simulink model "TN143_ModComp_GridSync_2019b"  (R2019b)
settings: Solver=VariableStepAuto  StartTime=0.0  StopTime=0.1  RelTol=1e-3
model workspace (MAT data in the model file):
  CTRLPERIOD = 5e-05
  global_can_baud_rate = 1000000
  global_cycle_delay = 1e-05
  global_ip_addresses : object (value not decoded)
undefined symbols (not defined in the file): A, AXI4, C, code, HLS, N, Stream, xc7z030fbg676
libraries: ModelComposer x102

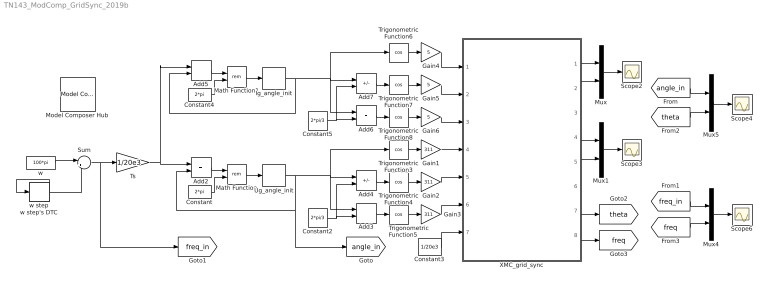
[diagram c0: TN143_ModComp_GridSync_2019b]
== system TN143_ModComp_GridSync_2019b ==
  Add{2..3,5..6} (4 alike) : Sum
  Add4 : Sum  Inputs=+-
  Add7 : Sum  Inputs=+-
  Constant : Constant  Value=2*pi  OutDataTypeStr=single
  Constant2 : Constant  Value=2*pi/3  OutDataTypeStr=single
  Constant3 : Constant  Value=1/20e3  OutDataTypeStr=single
  Constant4 : Constant  Value=2*pi  OutDataTypeStr=single
  Constant5 : Constant  Value=2*pi/3  OutDataTypeStr=single
  Gain1 : Gain  Gain=311
  Gain2 : Gain  Gain=311
  Gain3 : Gain  Gain=311
  Gain4 : Gain  Gain=5
  Gain5 : Gain  Gain=5
  Gain6 : Gain  Gain=5
  Ig_angle_init : Delay  DelayLength=1  InitialCondition=pi/2-pi/3
  Math Function : Math  Operator=rem
  Math Function1 : Math  Operator=rem
  Model Composer Hub : ModelComposer/Model Composer Hub  CodeGeneration=off  SubsystemName=XMC_grid_sync  TargetDirectory=C:/XMC/TN143/generated/code  ExportType=HLS C++ code  IpVendor=xilinx.com  IpLibrary=hls  IpVersion=1.0  IpHWLanguage=Verilog  AieCompilerOptions={}  CreateTestbench=off  TestbenchStackSize=10  RunAieSim=off  AieSimTimeout=50000  LaunchVitisAnalyzer=off  RunX86Sim=off  X86SimTimeout=10  ProjDevice=xc7z030fbg676-3  ProjDevicePart=xc7z030fbg676-3  SamplePeriod=-1  ClockFrequency=250  DataPathParallelism=1
  Mux{,1,4..5} (4 alike) : Mux  Inputs=2
  Scope{2..4,6} (4 alike) : Scope
  Sum : Sum  Inputs=|++
  Trigonometric Function{3..8} (6 alike) : Trigonometry  Operator=cos
  Ts : Gain  Gain=1/20e3
  Ug_angle_init : Delay  DelayLength=1  InitialCondition=0
  XMC_grid_sync : Subsystem  mask{PLL_KP=5, PLL_KI=2, FREQ=50}
      mask prompts: PLL_KP "PLL kp"; PLL_KI "PLL ki"; FREQ "PLL frequency(Hz)"
  w : Constant  Value=100*pi  OutDataTypeStr=single  SampleTime=1/20e3
  w step : Step  Time=0.02  After=10*pi
  w step's DTC : DataTypeConversion  OutDataTypeStr=single
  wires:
  Trigonometric Function4/1 -> Gain2/1
  Add2/1 -> Math Function/1
  Trigonometric Function3/1 -> Gain1/1
  Gain1/1 -> XMC_grid_sync/4(Ug_A)
  Gain3/1 -> XMC_grid_sync/6(Ug_C)
  Gain2/1 -> XMC_grid_sync/5(Ug_B)
  Constant2/1 -> Add4/2, Add3/2
  Add4/1 -> Trigonometric Function4/1
  Add3/1 -> Trigonometric Function5/1
  Math Function/1 -> Ug_angle_init/1
  Constant/1 -> Math Function/2
  Trigonometric Function5/1 -> Gain3/1
  Constant3/1 -> XMC_grid_sync/7(Ts)
  Gain6/1 -> XMC_grid_sync/3(Ig_C)
  Gain5/1 -> XMC_grid_sync/2(Ig_B)
  Gain4/1 -> XMC_grid_sync/1(Ig_A)
  XMC_grid_sync/1(Ig_d) -> Mux/1
  XMC_grid_sync/2(Ig_q) -> Mux/2
  Mux/1 -> Scope2/1
  XMC_grid_sync/4(Ug_d) -> Mux1/1
  XMC_grid_sync/5(Ug_q) -> Mux1/2
  Mux1/1 -> Scope3/1
  Ts/1 -> Add5/1, Add2/1
  Trigonometric Function8/1 -> Gain6/1
  Ig_angle_init/1 -> Trigonometric Function6/1, Add7/1, Add6/1, Add5/2
  Constant5/1 -> Add7/2, Add6/2
  Add7/1 -> Trigonometric Function7/1
  Constant4/1 -> Math Function1/2
  Add6/1 -> Trigonometric Function8/1
  Add5/1 -> Math Function1/1
  Trigonometric Function7/1 -> Gain5/1
  Trigonometric Function6/1 -> Gain4/1
  Math Function1/1 -> Ig_angle_init/1
  w/1 -> Sum/1
  Sum/1 -> Ts/1, [freq_in]
  Ug_angle_init/1 -> Trigonometric Function3/1, Add4/1, Add3/1, [angle_in], Add2/2
  XMC_grid_sync/7(theta) -> [theta]
  XMC_grid_sync/8(freq) -> [freq]
  [freq_in] -> Mux4/1
  [freq] -> Mux4/2
  [angle_in] -> Mux5/1
  [theta] -> Mux5/2
  Mux4/1 -> Scope6/1
  Mux5/1 -> Scope4/1
  w step/1 -> w step's DTC/1
  w step's DTC/1 -> Sum/2

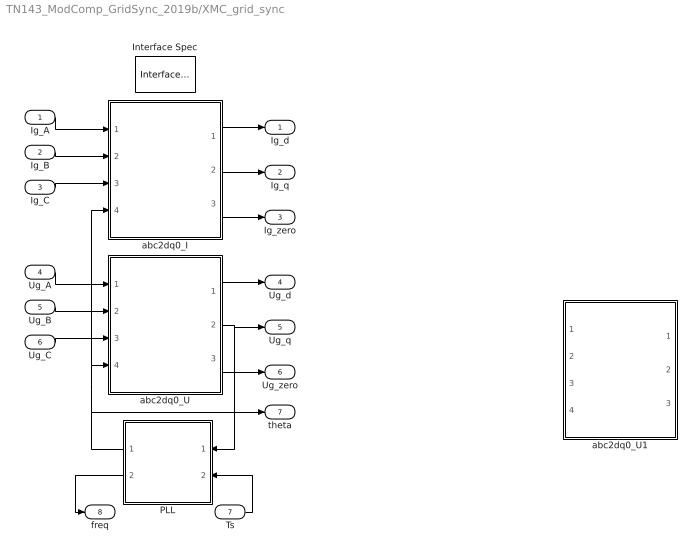
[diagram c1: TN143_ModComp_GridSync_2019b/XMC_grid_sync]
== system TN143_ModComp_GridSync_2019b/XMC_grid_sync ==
  Ig_A : Inport  OutDataTypeStr=single
  Ig_B : Inport  Port=2  OutDataTypeStr=single
  Ig_C : Inport  Port=3  OutDataTypeStr=single
  Ug_A : Inport  Port=4  OutDataTypeStr=single
  Ug_B : Inport  Port=5  OutDataTypeStr=single
  Ug_C : Inport  Port=6  OutDataTypeStr=single
  Ts : Inport  Port=7  OutDataTypeStr=single
  Interface Spec : ModelComposer/Interface Spec  Return=No block-level I/O protocol@@  InportInterfaces={'AXI4-Stream@@@N/A@N/A', 'AXI4-Stream@@@N/A@N/A', 'AXI4-Stream@@@N/A@N/A', 'AXI4-Stream@@@N/A@N/A', 'AXI4-Stream@@@N/A@N/A', 'AXI4-Stream@@@N/A@N/A', 'AXI4-Stream@@@N/A@N/A'}  InportHandles={1.164000122070312500e+03, 1.165000122070312500e+03, 1.166000122070312500e+03, 1.167000122070312500e+03, 1.168000122070312500e+03, 1.169000122070312500e+03, 1.170000122070312500e+03}  InportNames={'Ig_A', 'Ig_B', 'Ig_C', 'Ug_A', 'Ug_B', 'Ug_C', 'Ts'}  OutportInterfaces={'AXI4-Stream@@@N/A@N/A', 'AXI4-Stream@@@N/A@N/A', 'AXI4-Stream@@@N/A@N/A', 'AXI4-Stream@@@N/A@N/A', 'AXI4-Stream@@@N/A@N/A', 'AXI4-Stream@@@N/A@N/A', 'AXI4-Stream@@@N/A@N/A', 'Default@@@N/A@N/A'}  OutportHandles={1.505000366210937500e+03, 1.506000122070312500e+03, 1.507000122070312500e+03, 1.508000122070312500e+03, 1.509000122070312500e+03, 1.510000122070312500e+03, 1.511000122070312500e+03, 1.512000122070312500e+03}  OutportNames={'Ig_d', 'Ig_q', 'Ig_zero', 'Ug_d', 'Ug_q', 'Ug_zero', 'theta', 'freq'}  Mode=No block-level I/O protocol  InName1=Ig_A  InMode1=AXI4-Stream  InVFormat1=N/A  InVComponent1=N/A  InName2=Ig_B  InMode2=AXI4-Stream  InVFormat2=N/A  InVComponent2=N/A  InName3=Ig_C  InMode3=AXI4-Stream  InVFormat3=N/A  InVComponent3=N/A  InName4=Ug_A  InMode4=AXI4-Stream  InVFormat4=N/A  InVComponent4=N/A  InName5=Ug_B  InMode5=AXI4-Stream  InVFormat5=N/A  InVComponent5=N/A  InName6=Ug_C  InMode6=AXI4-Stream  InVFormat6=N/A  InVComponent6=N/A  InName7=Ts  InMode7=AXI4-Stream  InVFormat7=N/A  InVComponent7=N/A  InName8=CLOCK_period  InMode8=Constant  InVFormat8=N/A  InVComponent8=N/A  OutName1=Ig_d  OutMode1=AXI4-Stream  OutVFormat1=N/A  OutVComponent1=N/A  OutName2=Ig_q  OutMode2=AXI4-Stream  OutVFormat2=N/A  OutVComponent2=N/A  OutName3=Ig_zero  OutMode3=AXI4-Stream  OutVFormat3=N/A  OutVComponent3=N/A  OutName4=Ug_d  OutMode4=AXI4-Stream  OutVFormat4=N/A  OutVComponent4=N/A  OutName5=Ug_q  OutMode5=AXI4-Stream  OutVFormat5=N/A  OutVComponent5=N/A  OutName6=Ug_zero  OutMode6=AXI4-Stream  OutVFormat6=N/A  OutVComponent6=N/A  OutName7=theta  OutMode7=AXI4-Stream  OutVFormat7=N/A  OutVComponent7=N/A  OutName8=freq  OutMode8=Default  OutVFormat8=N/A  OutVComponent8=N/A
  PLL : Subsystem
  abc2dq0_I : Subsystem
  abc2dq0_U : Subsystem
  abc2dq0_U1 : Subsystem  Commented=on
  Ig_d : Outport
  Ig_q : Outport  Port=2
  Ig_zero : Outport  Port=3
  Ug_d : Outport  Port=4
  Ug_q : Outport  Port=5
  Ug_zero : Outport  Port=6
  theta : Outport  Port=7
  freq : Outport  Port=8
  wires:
  Ug_A/1 -> abc2dq0_U/1(A)
  Ig_B/1 -> abc2dq0_I/2(B)
  abc2dq0_I/3(zero) -> Ig_zero/1
  abc2dq0_I/2(q) -> Ig_q/1
  Ig_C/1 -> abc2dq0_I/3(C)
  abc2dq0_U/3(zero) -> Ug_zero/1
  Ug_B/1 -> abc2dq0_U/2(B)
  Ig_A/1 -> abc2dq0_I/1(A)
  abc2dq0_U/1(d) -> Ug_d/1
  Ug_C/1 -> abc2dq0_U/3(C)
  abc2dq0_I/1(d) -> Ig_d/1
  abc2dq0_U/2(q) -> Ug_q/1, PLL/1(err)
  PLL/1(theta) -> theta/1, abc2dq0_U/4(theta), abc2dq0_I/4(theta)
  Ts/1 -> PLL/2(Ts)
  PLL/2(freq) -> freq/1

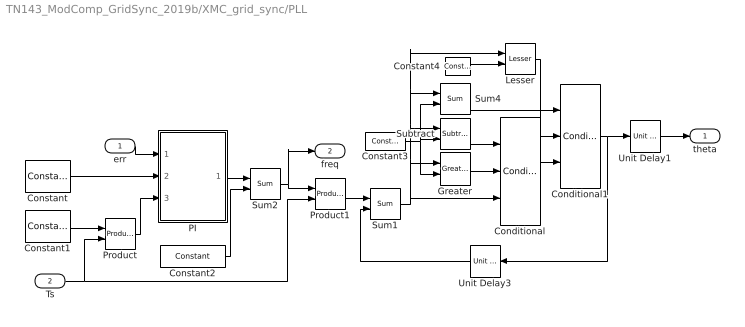
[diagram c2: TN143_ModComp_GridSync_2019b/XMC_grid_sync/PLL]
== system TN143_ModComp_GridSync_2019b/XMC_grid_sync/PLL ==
  err : Inport
  Ts : Inport  Port=2
  Conditional : ModelComposer/Conditional  Condition=C ~= 0  Threshold=0.00
  Conditional1 : ModelComposer/Conditional  Condition=C ~= 0  Threshold=0.00
  Constant : ModelComposer/Constant  Value=PLL_KP  SampleTime=-1  OutDataType=single  TypeExp=''  Signedness=Signed  WordLength=16  FractionalLength=0  RoundingMode=Truncation to minus infinity  OverflowMode=Wrap around
  Constant1 : ModelComposer/Constant  Value=PLL_KI  SampleTime=-1  OutDataType=single  TypeExp=''  Signedness=Signed  WordLength=16  FractionalLength=0  RoundingMode=Truncation to minus infinity  OverflowMode=Wrap around
  Constant2 : ModelComposer/Constant  Value=2*pi*FREQ  SampleTime=-1  OutDataType=single  TypeExp=''  Signedness=Signed  WordLength=16  FractionalLength=0  RoundingMode=Truncation to minus infinity  OverflowMode=Wrap around
  Constant3 : ModelComposer/Constant  Value=2*pi  SampleTime=-1  OutDataType=single  TypeExp=''  Signedness=Signed  WordLength=16  FractionalLength=0  RoundingMode=Truncation to minus infinity  OverflowMode=Wrap around
  Constant4 : ModelComposer/Constant  Value=0  SampleTime=-1  OutDataType=single  TypeExp=''  Signedness=Signed  WordLength=16  FractionalLength=0  RoundingMode=Truncation to minus infinity  OverflowMode=Wrap around
  Greater : ModelComposer/Greater
  Lesser : ModelComposer/Lesser
  PI : Subsystem
  Product : ModelComposer/Product
  Product1 : ModelComposer/Product
  Subtract : ModelComposer/Subtract
  Sum1 : ModelComposer/Sum
  Sum2 : ModelComposer/Sum
  Sum4 : ModelComposer/Sum
  Unit Delay1 : ModelComposer/Unit Delay  InitialCondition=0
  Unit Delay3 : ModelComposer/Unit Delay  InitialCondition=0
  theta : Outport
  freq : Outport  Port=2
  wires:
  Constant2/1 -> Sum2/2
  Conditional1/1 -> Unit Delay3/1, Unit Delay1/1
  Ts/1 -> Product1/2, Product/2
  Subtract/1 -> Conditional/1
  Constant4/1 -> Lesser/2
  Sum2/1 -> freq/1, Product1/1
  Greater/1 -> Conditional/2
  Constant1/1 -> Product/1
  Constant3/1 -> Greater/2, Subtract/2, Sum4/2
  Unit Delay3/1 -> Sum1/2
  Conditional/1 -> Conditional1/3
  Lesser/1 -> Conditional1/2
  PI/1(Out) -> Sum2/1
  Sum1/1 -> Conditional/3, Greater/1, Subtract/1, Sum4/1, Lesser/1
  Product1/1 -> Sum1/1
  Constant/1 -> PI/2(kp)
  Unit Delay1/1 -> theta/1
  Product/1 -> PI/3(ki)
  Sum4/1 -> Conditional1/1
  err/1 -> PI/1(err)

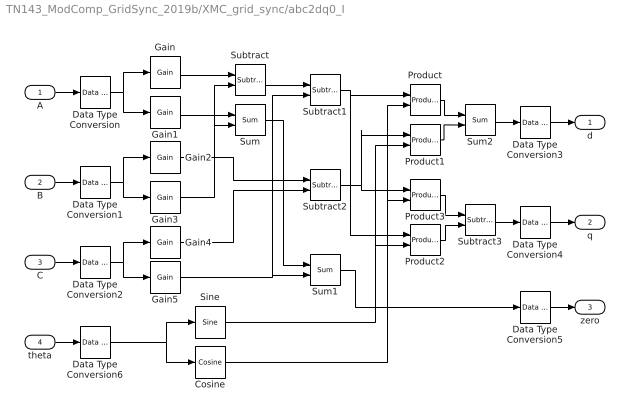
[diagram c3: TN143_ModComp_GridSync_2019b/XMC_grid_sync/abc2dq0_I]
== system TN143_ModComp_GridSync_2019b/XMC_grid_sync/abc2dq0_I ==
  A : Inport  OutDataTypeStr=single
  B : Inport  Port=2  OutDataTypeStr=single
  C : Inport  Port=3  OutDataTypeStr=single
  theta : Inport  Port=4  OutDataTypeStr=single
  Cosine : ModelComposer/Cosine
  Data Type Conversion : ModelComposer/Data Type Conversion  OutDataType=fixed  TypeExp=''  Signedness=Signed  WordLength=32  FractionalLength=16  RoundingMode=Truncation to minus infinity  OverflowMode=Wrap around
  Data Type Conversion1 : ModelComposer/Data Type Conversion  OutDataType=fixed  TypeExp=''  Signedness=Signed  WordLength=32  FractionalLength=16  RoundingMode=Truncation to minus infinity  OverflowMode=Wrap around
  Data Type Conversion2 : ModelComposer/Data Type Conversion  OutDataType=fixed  TypeExp=''  Signedness=Signed  WordLength=32  FractionalLength=16  RoundingMode=Truncation to minus infinity  OverflowMode=Wrap around
  Data Type Conversion3 : ModelComposer/Data Type Conversion  OutDataType=single  TypeExp=''  Signedness=Signed  WordLength=32  FractionalLength=16  RoundingMode=Truncation to minus infinity  OverflowMode=Wrap around
  Data Type Conversion4 : ModelComposer/Data Type Conversion  OutDataType=single  TypeExp=''  Signedness=Signed  WordLength=32  FractionalLength=16  RoundingMode=Truncation to minus infinity  OverflowMode=Wrap around
  Data Type Conversion5 : ModelComposer/Data Type Conversion  OutDataType=single  TypeExp=''  Signedness=Signed  WordLength=32  FractionalLength=16  RoundingMode=Truncation to minus infinity  OverflowMode=Wrap around
  Data Type Conversion6 : ModelComposer/Data Type Conversion  OutDataType=fixed  TypeExp=''  Signedness=Signed  WordLength=16  FractionalLength=12  RoundingMode=Truncation to minus infinity  OverflowMode=Wrap around
  Gain : ModelComposer/Gain  Gain=2/3  OutDataType=single  TypeExp=''  Signedness=Signed  WordLength=16  FractionalLength=0  RoundingMode=Truncation to minus infinity  OverflowMode=Wrap around  OutputTypeAsInput=on
  Gain1 : ModelComposer/Gain  Gain=1/3  OutDataType=single  TypeExp=''  Signedness=Signed  WordLength=16  FractionalLength=0  RoundingMode=Truncation to minus infinity  OverflowMode=Wrap around  OutputTypeAsInput=on
  Gain2 : ModelComposer/Gain  Gain=sqrt(3)/3  OutDataType=single  TypeExp=''  Signedness=Signed  WordLength=16  FractionalLength=0  RoundingMode=Truncation to minus infinity  OverflowMode=Wrap around  OutputTypeAsInput=on
  Gain3 : ModelComposer/Gain  Gain=1/3  OutDataType=single  TypeExp=''  Signedness=Signed  WordLength=16  FractionalLength=0  RoundingMode=Truncation to minus infinity  OverflowMode=Wrap around  OutputTypeAsInput=on
  Gain4 : ModelComposer/Gain  Gain=sqrt(3)/3  OutDataType=single  TypeExp=''  Signedness=Signed  WordLength=16  FractionalLength=0  RoundingMode=Truncation to minus infinity  OverflowMode=Wrap around  OutputTypeAsInput=on
  Gain5 : ModelComposer/Gain  Gain=1/3  OutDataType=single  TypeExp=''  Signedness=Signed  WordLength=16  FractionalLength=0  RoundingMode=Truncation to minus infinity  OverflowMode=Wrap around  OutputTypeAsInput=on
  Product{,1..3} (4 alike) : ModelComposer/Product
  Sine : ModelComposer/Sine
  Subtract{,1..3} (4 alike) : ModelComposer/Subtract
  Sum : ModelComposer/Sum
  Sum1 : ModelComposer/Sum
  Sum2 : ModelComposer/Sum
  d : Outport  OutDataTypeStr=single
  q : Outport  Port=2  OutDataTypeStr=single
  zero : Outport  Port=3  OutDataTypeStr=single
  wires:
  Product2/1 -> Subtract3/2
  Subtract1/1 -> Product2/1, Product/1
  Data Type Conversion4/1 -> q/1
  Gain1/1 -> Sum/1
  A/1 -> Data Type Conversion/1
  Data Type Conversion/1 -> Gain/1, Gain1/1
  Gain/1 -> Subtract/1
  Sum2/1 -> Data Type Conversion3/1
  Product1/1 -> Sum2/2
  Sum/1 -> Sum1/1
  Data Type Conversion3/1 -> d/1
  Subtract3/1 -> Data Type Conversion4/1
  Gain4/1 -> Subtract2/2
  Subtract/1 -> Subtract1/1
  Product/1 -> Sum2/1
  Data Type Conversion2/1 -> Gain4/1, Gain5/1
  B/1 -> Data Type Conversion1/1
  Cosine/1 -> Product/2, Product3/2
  Subtract2/1 -> Product1/1, Product3/1
  Product3/1 -> Subtract3/1
  Data Type Conversion6/1 -> Cosine/1, Sine/1
  Gain3/1 -> Subtract/2, Sum/2
  theta/1 -> Data Type Conversion6/1
  Gain2/1 -> Subtract2/1
  Data Type Conversion1/1 -> Gain2/1, Gain3/1
  Sum1/1 -> Data Type Conversion5/1
  C/1 -> Data Type Conversion2/1
  Gain5/1 -> Sum1/2, Subtract1/2
  Sine/1 -> Product1/2, Product2/2
  Data Type Conversion5/1 -> zero/1

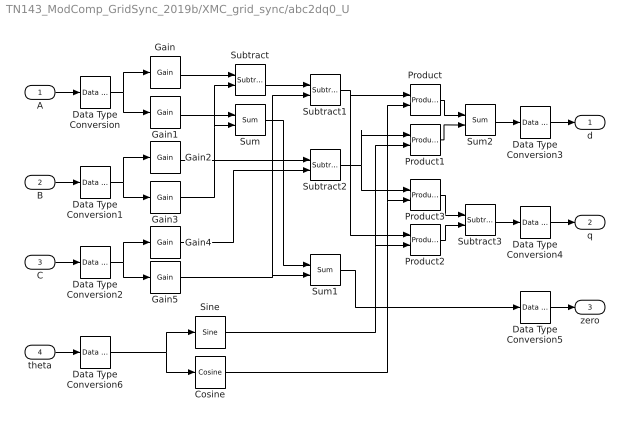
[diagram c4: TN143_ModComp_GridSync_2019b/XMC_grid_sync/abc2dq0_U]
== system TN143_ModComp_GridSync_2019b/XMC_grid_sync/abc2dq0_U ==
  A : Inport  OutDataTypeStr=single
  B : Inport  Port=2  OutDataTypeStr=single
  C : Inport  Port=3  OutDataTypeStr=single
  theta : Inport  Port=4  OutDataTypeStr=single
  Cosine : ModelComposer/Cosine
  Data Type Conversion : ModelComposer/Data Type Conversion  OutDataType=fixed  TypeExp=''  Signedness=Signed  WordLength=32  FractionalLength=16  RoundingMode=Truncation to minus infinity  OverflowMode=Wrap around
  Data Type Conversion1 : ModelComposer/Data Type Conversion  OutDataType=fixed  TypeExp=''  Signedness=Signed  WordLength=32  FractionalLength=16  RoundingMode=Truncation to minus infinity  OverflowMode=Wrap around
  Data Type Conversion2 : ModelComposer/Data Type Conversion  OutDataType=fixed  TypeExp=''  Signedness=Signed  WordLength=32  FractionalLength=16  RoundingMode=Truncation to minus infinity  OverflowMode=Wrap around
  Data Type Conversion3 : ModelComposer/Data Type Conversion  OutDataType=single  TypeExp=''  Signedness=Signed  WordLength=32  FractionalLength=16  RoundingMode=Truncation to minus infinity  OverflowMode=Wrap around
  Data Type Conversion4 : ModelComposer/Data Type Conversion  OutDataType=single  TypeExp=''  Signedness=Signed  WordLength=32  FractionalLength=16  RoundingMode=Truncation to minus infinity  OverflowMode=Wrap around
  Data Type Conversion5 : ModelComposer/Data Type Conversion  OutDataType=single  TypeExp=''  Signedness=Signed  WordLength=32  FractionalLength=16  RoundingMode=Truncation to minus infinity  OverflowMode=Wrap around
  Data Type Conversion6 : ModelComposer/Data Type Conversion  OutDataType=fixed  TypeExp=''  Signedness=Signed  WordLength=16  FractionalLength=12  RoundingMode=Truncation to minus infinity  OverflowMode=Wrap around
  Gain : ModelComposer/Gain  Gain=2/3  OutDataType=single  TypeExp=''  Signedness=Signed  WordLength=16  FractionalLength=0  RoundingMode=Truncation to minus infinity  OverflowMode=Wrap around  OutputTypeAsInput=on
  Gain1 : ModelComposer/Gain  Gain=1/3  OutDataType=single  TypeExp=''  Signedness=Signed  WordLength=16  FractionalLength=0  RoundingMode=Truncation to minus infinity  OverflowMode=Wrap around  OutputTypeAsInput=on
  Gain2 : ModelComposer/Gain  Gain=sqrt(3)/3  OutDataType=single  TypeExp=''  Signedness=Signed  WordLength=16  FractionalLength=0  RoundingMode=Truncation to minus infinity  OverflowMode=Wrap around  OutputTypeAsInput=on
  Gain3 : ModelComposer/Gain  Gain=1/3  OutDataType=single  TypeExp=''  Signedness=Signed  WordLength=16  FractionalLength=0  RoundingMode=Truncation to minus infinity  OverflowMode=Wrap around  OutputTypeAsInput=on
  Gain4 : ModelComposer/Gain  Gain=sqrt(3)/3  OutDataType=single  TypeExp=''  Signedness=Signed  WordLength=16  FractionalLength=0  RoundingMode=Truncation to minus infinity  OverflowMode=Wrap around  OutputTypeAsInput=on
  Gain5 : ModelComposer/Gain  Gain=1/3  OutDataType=single  TypeExp=''  Signedness=Signed  WordLength=16  FractionalLength=0  RoundingMode=Truncation to minus infinity  OverflowMode=Wrap around  OutputTypeAsInput=on
  Product{,1..3} (4 alike) : ModelComposer/Product
  Sine : ModelComposer/Sine
  Subtract{,1..3} (4 alike) : ModelComposer/Subtract
  Sum : ModelComposer/Sum
  Sum1 : ModelComposer/Sum
  Sum2 : ModelComposer/Sum
  d : Outport  OutDataTypeStr=single
  q : Outport  Port=2  OutDataTypeStr=single
  zero : Outport  Port=3  OutDataTypeStr=single
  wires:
  Data Type Conversion5/1 -> zero/1
  Sine/1 -> Product2/2, Product1/2
  Gain5/1 -> Subtract1/2, Sum1/2
  C/1 -> Data Type Conversion2/1
  Sum1/1 -> Data Type Conversion5/1
  Data Type Conversion1/1 -> Gain3/1, Gain2/1
  Gain2/1 -> Subtract2/1
  theta/1 -> Data Type Conversion6/1
  Gain3/1 -> Sum/2, Subtract/2
  Data Type Conversion6/1 -> Sine/1, Cosine/1
  Product3/1 -> Subtract3/1
  Subtract2/1 -> Product1/1, Product3/1
  Cosine/1 -> Product3/2, Product/2
  B/1 -> Data Type Conversion1/1
  Data Type Conversion2/1 -> Gain5/1, Gain4/1
  Product/1 -> Sum2/1
  Subtract/1 -> Subtract1/1
  Gain4/1 -> Subtract2/2
  Subtract3/1 -> Data Type Conversion4/1
  Data Type Conversion3/1 -> d/1
  Sum/1 -> Sum1/1
  Product1/1 -> Sum2/2
  Sum2/1 -> Data Type Conversion3/1
  Gain/1 -> Subtract/1
  Data Type Conversion/1 -> Gain1/1, Gain/1
  A/1 -> Data Type Conversion/1
  Gain1/1 -> Sum/1
  Data Type Conversion4/1 -> q/1
  Subtract1/1 -> Product/1, Product2/1
  Product2/1 -> Subtract3/2

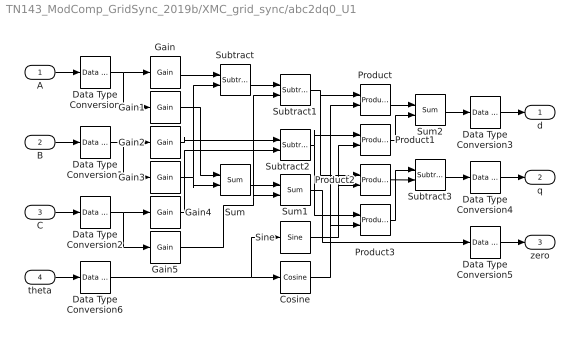
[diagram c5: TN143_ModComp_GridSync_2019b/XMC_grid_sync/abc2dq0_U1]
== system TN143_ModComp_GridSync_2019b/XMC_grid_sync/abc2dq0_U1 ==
  A : Inport  OutDataTypeStr=single
  B : Inport  Port=2  OutDataTypeStr=single
  C : Inport  Port=3  OutDataTypeStr=single
  theta : Inport  Port=4  OutDataTypeStr=single
  Cosine : ModelComposer/Cosine
  Data Type Conversion : ModelComposer/Data Type Conversion  OutDataType=fixed  TypeExp=''  Signedness=Signed  WordLength=32  FractionalLength=16  RoundingMode=Truncation to minus infinity  OverflowMode=Wrap around
  Data Type Conversion1 : ModelComposer/Data Type Conversion  OutDataType=fixed  TypeExp=''  Signedness=Signed  WordLength=32  FractionalLength=16  RoundingMode=Truncation to minus infinity  OverflowMode=Wrap around
  Data Type Conversion2 : ModelComposer/Data Type Conversion  OutDataType=fixed  TypeExp=''  Signedness=Signed  WordLength=32  FractionalLength=16  RoundingMode=Truncation to minus infinity  OverflowMode=Wrap around
  Data Type Conversion3 : ModelComposer/Data Type Conversion  OutDataType=single  TypeExp=''  Signedness=Signed  WordLength=32  FractionalLength=16  RoundingMode=Truncation to minus infinity  OverflowMode=Wrap around
  Data Type Conversion4 : ModelComposer/Data Type Conversion  OutDataType=single  TypeExp=''  Signedness=Signed  WordLength=32  FractionalLength=16  RoundingMode=Truncation to minus infinity  OverflowMode=Wrap around
  Data Type Conversion5 : ModelComposer/Data Type Conversion  OutDataType=single  TypeExp=''  Signedness=Signed  WordLength=32  FractionalLength=16  RoundingMode=Truncation to minus infinity  OverflowMode=Wrap around
  Data Type Conversion6 : ModelComposer/Data Type Conversion  OutDataType=fixed  TypeExp=''  Signedness=Signed  WordLength=16  FractionalLength=12  RoundingMode=Truncation to minus infinity  OverflowMode=Wrap around
  Gain : ModelComposer/Gain  Gain=2/3  OutDataType=single  TypeExp=''  Signedness=Signed  WordLength=16  FractionalLength=0  RoundingMode=Truncation to minus infinity  OverflowMode=Wrap around  OutputTypeAsInput=on
  Gain1 : ModelComposer/Gain  Gain=1/3  OutDataType=single  TypeExp=''  Signedness=Signed  WordLength=16  FractionalLength=0  RoundingMode=Truncation to minus infinity  OverflowMode=Wrap around  OutputTypeAsInput=on
  Gain2 : ModelComposer/Gain  Gain=sqrt(3)/3  OutDataType=single  TypeExp=''  Signedness=Signed  WordLength=16  FractionalLength=0  RoundingMode=Truncation to minus infinity  OverflowMode=Wrap around  OutputTypeAsInput=on
  Gain3 : ModelComposer/Gain  Gain=1/3  OutDataType=single  TypeExp=''  Signedness=Signed  WordLength=16  FractionalLength=0  RoundingMode=Truncation to minus infinity  OverflowMode=Wrap around  OutputTypeAsInput=on
  Gain4 : ModelComposer/Gain  Gain=sqrt(3)/3  OutDataType=single  TypeExp=''  Signedness=Signed  WordLength=16  FractionalLength=0  RoundingMode=Truncation to minus infinity  OverflowMode=Wrap around  OutputTypeAsInput=on
  Gain5 : ModelComposer/Gain  Gain=1/3  OutDataType=single  TypeExp=''  Signedness=Signed  WordLength=16  FractionalLength=0  RoundingMode=Truncation to minus infinity  OverflowMode=Wrap around  OutputTypeAsInput=on
  Product{,1..3} (4 alike) : ModelComposer/Product
  Sine : ModelComposer/Sine
  Subtract{,1..3} (4 alike) : ModelComposer/Subtract
  Sum : ModelComposer/Sum
  Sum1 : ModelComposer/Sum
  Sum2 : ModelComposer/Sum
  d : Outport  OutDataTypeStr=single
  q : Outport  Port=2  OutDataTypeStr=single
  zero : Outport  Port=3  OutDataTypeStr=single
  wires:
  Data Type Conversion5/1 -> zero/1
  Sine/1 -> Product1/2, Product2/2
  Gain5/1 -> Sum1/2, Subtract1/2
  C/1 -> Data Type Conversion2/1
  Sum1/1 -> Data Type Conversion5/1
  Data Type Conversion1/1 -> Gain2/1, Gain3/1
  Gain2/1 -> Subtract2/1
  theta/1 -> Data Type Conversion6/1
  Gain3/1 -> Sum/2, Subtract/2
  Data Type Conversion6/1 -> Sine/1, Cosine/1
  Product3/1 -> Subtract3/1
  Subtract2/1 -> Product3/1, Product1/1
  Cosine/1 -> Product3/2, Product/2
  B/1 -> Data Type Conversion1/1
  Data Type Conversion2/1 -> Gain4/1, Gain5/1
  Product/1 -> Sum2/1
  Subtract/1 -> Subtract1/1
  Gain4/1 -> Subtract2/2
  Subtract3/1 -> Data Type Conversion4/1
  Data Type Conversion3/1 -> d/1
  Sum/1 -> Sum1/1
  Product1/1 -> Sum2/2
  Sum2/1 -> Data Type Conversion3/1
  Gain/1 -> Subtract/1
  Data Type Conversion/1 -> Gain/1, Gain1/1
  A/1 -> Data Type Conversion/1
  Gain1/1 -> Sum/1
  Data Type Conversion4/1 -> q/1
  Subtract1/1 -> Product2/1, Product/1
  Product2/1 -> Subtract3/2

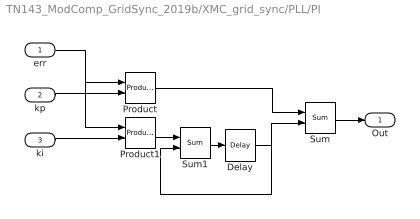
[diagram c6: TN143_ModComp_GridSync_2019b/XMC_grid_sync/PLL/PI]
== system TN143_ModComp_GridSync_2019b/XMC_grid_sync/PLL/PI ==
  err : Inport
  kp : Inport  Port=2
  ki : Inport  Port=3
  Delay : ModelComposer/Delay  Latency=1
  Product : ModelComposer/Product
  Product1 : ModelComposer/Product
  Sum : ModelComposer/Sum
  Sum1 : ModelComposer/Sum
  Out : Outport
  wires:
  Delay/1 -> Sum/2, Sum1/2
  Sum1/1 -> Delay/1
  Product1/1 -> Sum1/1
  Product/1 -> Sum/1
  Sum/1 -> Out/1
  ki/1 -> Product1/2
  kp/1 -> Product/2
  err/1 -> Product/1, Product1/1
